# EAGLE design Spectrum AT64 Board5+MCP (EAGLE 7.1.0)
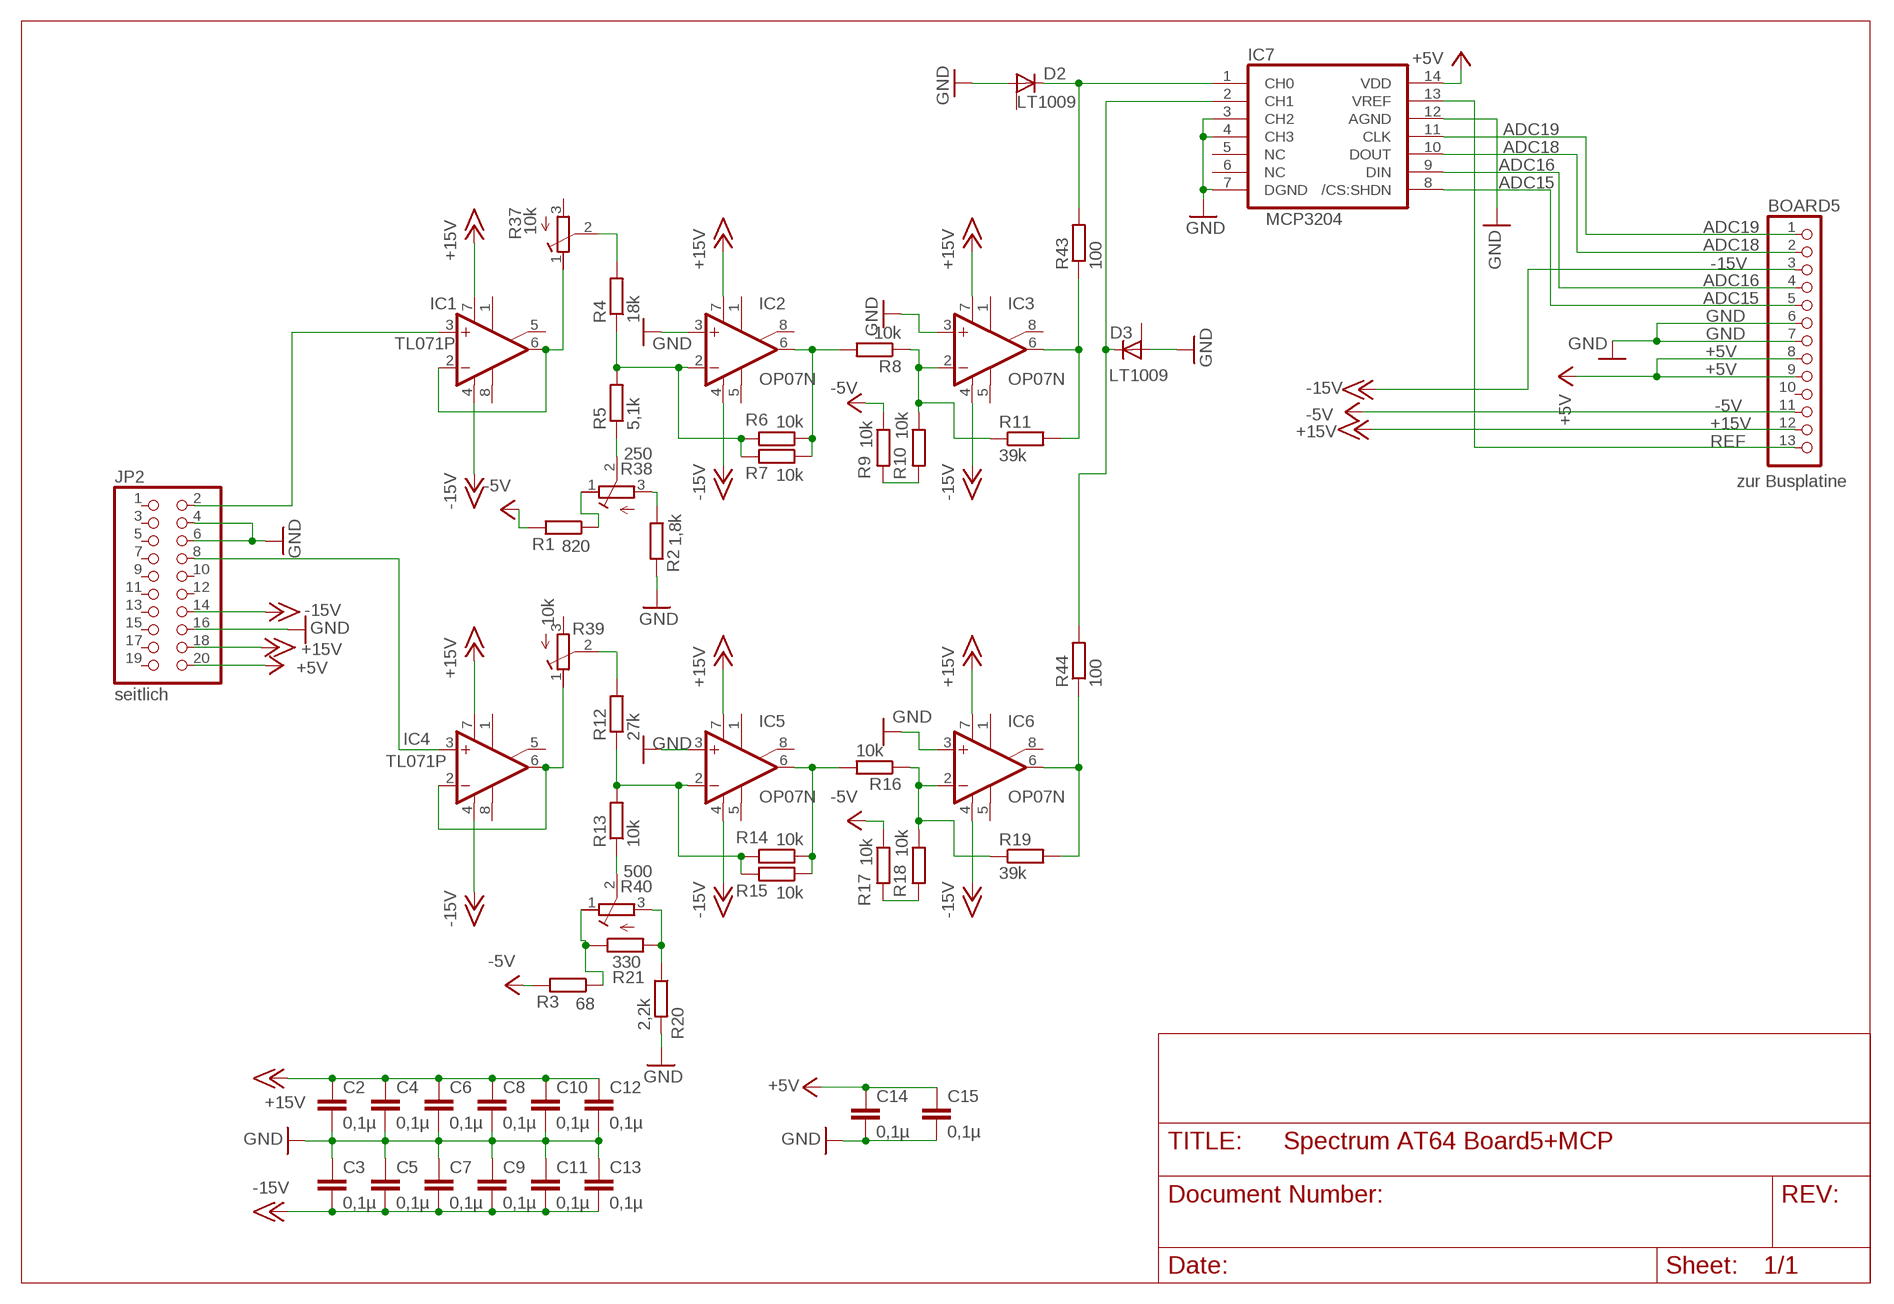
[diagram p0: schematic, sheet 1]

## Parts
BOARD5  zur Busplatine  PINHD-1X13_2.54-90°  [1X13/90]
C2  0,1µ  C-EU050-025X075  [C050-025X075]
C3  0,1µ  C-EUC0805  [C0805]
C4  0,1µ  C-EU050-025X075  [C050-025X075]
C5  0,1µ  C-EUC0805  [C0805]
C6  0,1µ  C-EU050-025X075  [C050-025X075]
C7  0,1µ  C-EU050-025X075  [C050-025X075]
C8  0,1µ  C-EU050-025X075  [C050-025X075]
C9  0,1µ  C-EU050-025X075  [C050-025X075]
C10  0,1µ  C-EU050-025X075  [C050-025X075]
C11  0,1µ  C-EU050-025X075  [C050-025X075]
C12  0,1µ  C-EU050-025X075  [C050-025X075]
C13  0,1µ  C-EU050-025X075  [C050-025X075]
C14  0,1µ  C-EU050-025X075  [C050-025X075]
C15  0,1µ  C-EU050-025X075  [C050-025X075]
D2  LT1009  [LT1009]
D3  LT1009  [LT1009]
IC1  TL071P  [DIL08]
IC2  OP07N  [DIL08]
IC3  OP07N  [DIL08]
IC4  TL071P  [DIL08]
IC5  OP07N  [DIL08]
IC6  OP07N  [DIL08]
IC7  MCP3204  [DIL14]
JP2  seitlich  PINHD-2X10_2.54-90°  [2X10/90]
R1  820  WIDERSTAND_10  [207.10]
R2  1,8k  WIDERSTAND_10  [207.10]
R3  68  WIDERSTAND_10  [207.10]
R4  18k  WIDERSTAND_10  [207.10]
R5  5,1k  WIDERSTAND_10  [207.10]
R6  10k  WIDERSTAND_10  [207.10]
R7  10k  WIDERSTAND_10  [207.10]
R8  10k  WIDERSTAND_10  [207.10]
R9  10k  WIDERSTAND_10  [207.10]
R10  10k  WIDERSTAND_10  [207.10]
R11  39k  WIDERSTAND_10  [207.10]
R12  27k  WIDERSTAND_10  [207.10]
R13  10k  WIDERSTAND_10  [207.10]
R14  10k  WIDERSTAND_10  [207.10]
R15  10k  WIDERSTAND_10  [207.10]
R16  10k  WIDERSTAND_10  [207.10]
R17  10k  WIDERSTAND_10  [207.10]
R18  10k  WIDERSTAND_10  [207.10]
R19  39k  WIDERSTAND_10  [207.10]
R20  2,2k  WIDERSTAND_10  [207.10]
R21  330  WIDERSTAND_10  [207.10]
R37  10k  R-TRIMM43P  [RTRIM43P]
R38  250  R-TRIMM43P  [RTRIM43P]
R39  10k  R-TRIMM43P  [RTRIM43P]
R40  500  R-TRIMM43P  [RTRIM43P]
R43  100  WIDERSTAND_10  [207.10]
R44  100  WIDERSTAND_10  [207.10]

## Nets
+5V: BOARD5.8 BOARD5.9 C14.1 C15.1 IC7.14(VDD) JP2.20
+15V: BOARD5.12 C2.1 C4.1 C6.1 C8.1 C10.1 C12.1 IC1.7(V+) IC2.7(V+) IC3.7(V+) IC4.7(V+) IC5.7(V+) IC6.7(V+) JP2.18
-5V: BOARD5.11 R1.2 R3.2 R9.1 R17.1
-15V: BOARD5.3 C3.2 C5.2 C7.2 C9.2 C11.2 C13.2 IC1.4(V-) IC2.4(V-) IC3.4(V-) IC4.4(V-) IC5.4(V-) IC6.4(V-) JP2.14
ADC15: BOARD5.5 IC7.8(/CS:SHDN)
ADC16: BOARD5.4 IC7.9(DIN)
ADC18: BOARD5.2 IC7.10(DOUT)
ADC19: BOARD5.1 IC7.11(CLK)
GND: BOARD5.6 BOARD5.7 C2.2 C3.1 C4.2 C5.1 C6.2 C7.1 C8.2 C9.1 C10.2 C11.1 C12.2 C13.1 C14.2 C15.2 D2.-(A) D3.-(A) IC2.3(+IN) IC3.3(+IN) IC5.3(+IN) IC6.3(+IN) IC7.3(CH2) IC7.4(CH3) IC7.7(DGND) IC7.12(AGND) JP2.4 JP2.6 JP2.16 R2.2 R20.2
N$1: R1.1 R38.1(A)
N$2: R2.1 R38.3(E)
N$3: R3.1 R21.1 R40.1(A)
N$4: R20.1 R21.2 R40.3(E)
N$6: IC1.3(+IN) JP2.2
N$7: IC1.2(-IN) IC1.6(OUT) R37.1(A)
N$8: R5.1 R38.2(S)
N$9: D3.+(C) IC7.2(CH1) R44.2
N$10: R4.2 R37.2(S)
N$11: IC2.6(OUT) R6.1 R7.1 R8.2
N$12: IC2.2(-IN) R4.1 R5.2 R6.2 R7.2
N$13: IC3.2(-IN) R8.1 R10.1 R11.1
N$14: R9.2 R10.2
N$15: IC3.6(OUT) R11.2 R43.1
N$16: IC4.3(+IN) JP2.8
N$17: D2.+(C) IC7.1(CH0) R43.2
N$18: IC4.2(-IN) IC4.6(OUT) R39.1(A)
N$19: R13.1 R40.2(S)
N$20: R12.2 R39.2(S)
N$21: IC5.6(OUT) R14.1 R15.1 R16.2
N$22: IC5.2(-IN) R12.1 R13.2 R14.2 R15.2
N$23: IC6.2(-IN) R16.1 R18.1 R19.1
N$24: R17.2 R18.2
N$25: IC6.6(OUT) R19.2 R44.1
REF: BOARD5.13 IC7.13(VREF)
Unconnected: BOARD5.10 D2.ADJ D3.ADJ IC1.1(ON1) IC1.5(ON2) IC1.8(OPT) IC2.1(ON1) IC2.5(OPT) IC2.8(ON2) IC3.1(ON1) IC3.5(OPT) IC3.8(ON2) IC4.1(ON1) IC4.5(ON2) IC4.8(OPT) IC5.1(ON1) IC5.5(OPT) IC5.8(ON2) IC6.1(ON1) IC6.5(OPT) IC6.8(ON2) IC7.5(NC) IC7.6(NC) JP2.1 JP2.3 JP2.5 JP2.7 JP2.9 JP2.10 JP2.11 JP2.12 JP2.13 JP2.15 JP2.17 JP2.19 R37.3(E) R39.3(E)

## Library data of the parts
BOARD5 = pinhead-2:PINHD-1X13: PIN HEADER
C2-C15 = rcl:C-EU: CAPACITOR, European symbol
D2 D3 = 1Eigene:LT1009
IC1 IC4 = linear:TL071: OP AMP
IC2 IC3 IC5 IC6 = linear:OP07*: OP AMP
IC7 = 1Eigene:MCP3204
JP2 = pinhead-2:PINHD-2X10: PIN HEADER
R1-R21 R43 R44 = 1Eigene:WIDERSTAND_10
R37-R40 = rcl:R-TRIMM: Trimm resistor

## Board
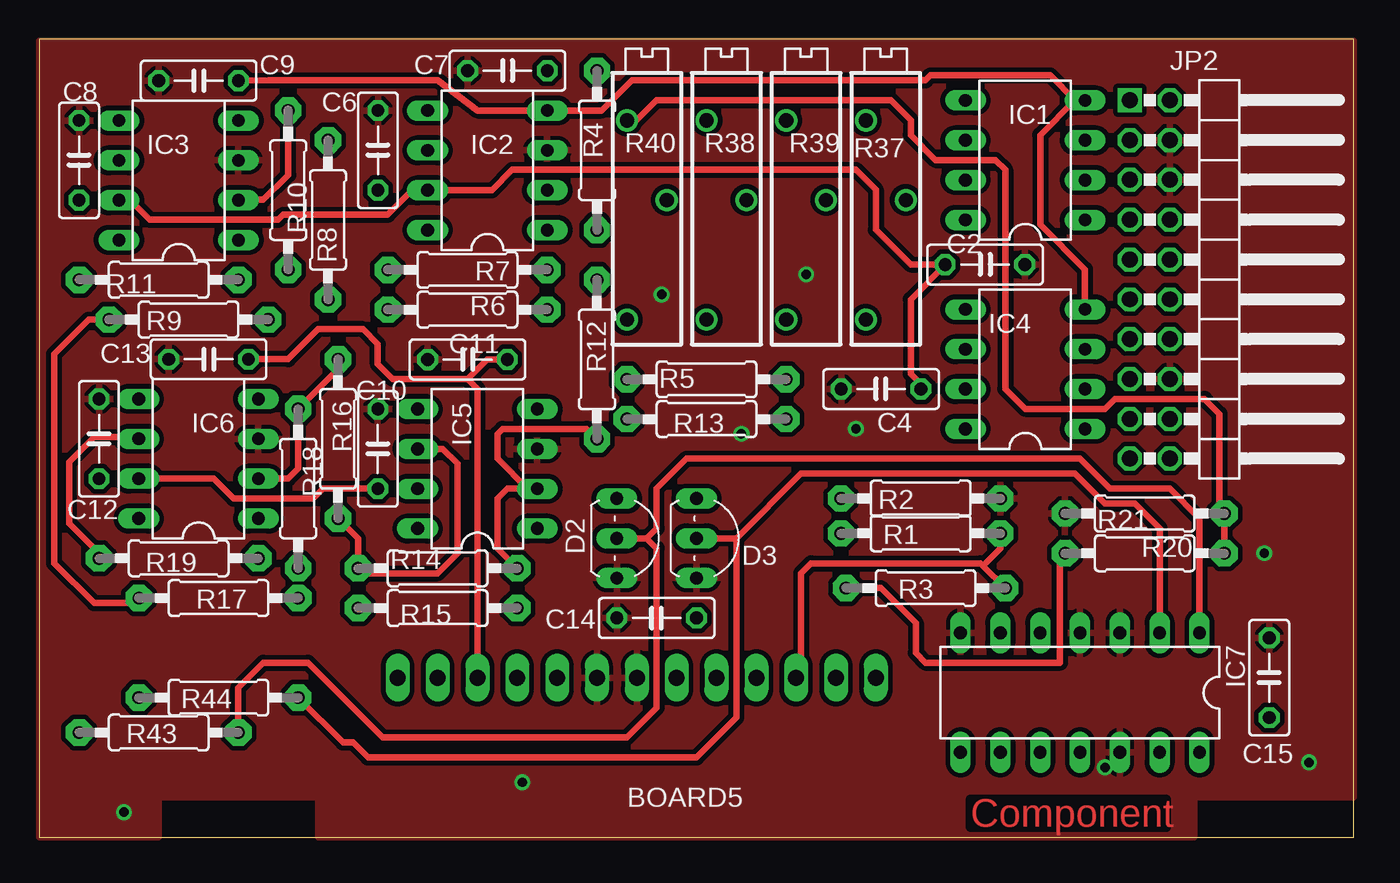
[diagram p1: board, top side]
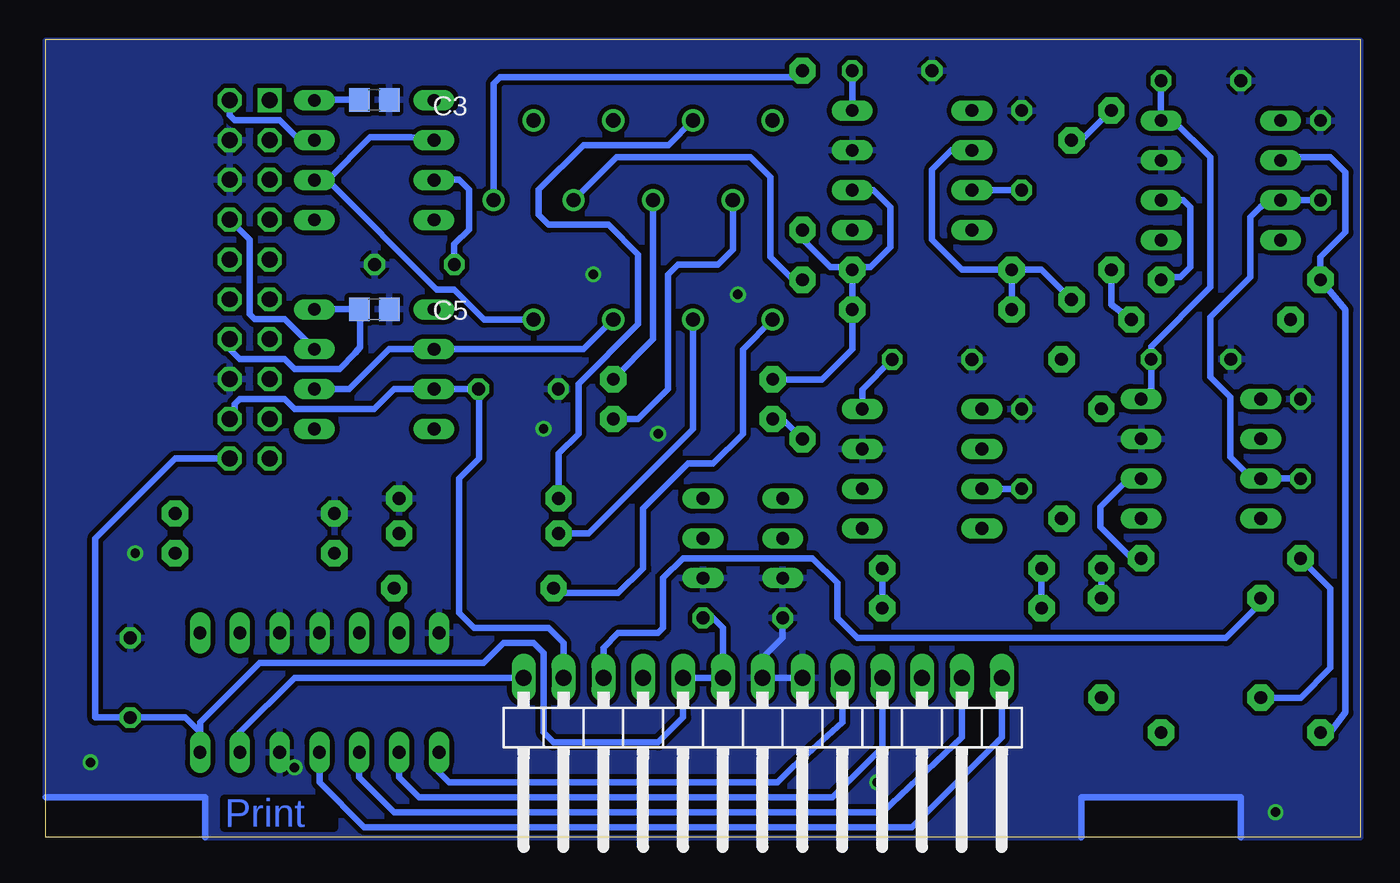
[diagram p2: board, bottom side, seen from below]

Size 83.8 x 50.88 mm. Coordinates in mm from the lower left corner, seen from the top.
Outline: 0,0 83.8,0 83.8,50.88 0,50.88 0,0
Copper layers (1*16): Top 0.035mm / dielectric 1.5mm / Bottom 0.035mm
Design rules "default *": minimum track width 0.4mm, minimum drill 0.6mm, track to track 0.3mm, track to pad 0.3mm, pad to pad 0.3mm, via to via 0.3mm, smd to smd 0.3mm, copper to edge 0mil, drill to drill 8mil, minimum pad ring 10mil, minimum via ring 8mil, stop-mask expansion 4mil, vias tented up to drill 0mil, thermal gap 10mil

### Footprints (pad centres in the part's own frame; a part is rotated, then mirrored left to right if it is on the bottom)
1X13/90 = drill 1.016 long: 1 -15.24,-3.81; 2 -12.7,-3.81; 3 -10.16,-3.81; 4 -7.62,-3.81; 5 -5.08,-3.81; 6 -2.54,-3.81; 7 0,-3.81; 8 2.54,-3.81; 9 5.08,-3.81; 10 7.62,-3.81; 11 10.16,-3.81; 12 12.7,-3.81; 13 15.24,-3.81
C050-025X075 = drill 0.813 octagon: 1 -2.54,0; 2 2.54,0
C0805 = smd 1.3 x 1.5: 1 -0.95,0; 2 0.95,0
LT1009 = drill 0.813 long: + 0,0; - 2.54,0; ADJ -2.54,0
DIL08 = drill 0.813 long: 1 -3.81,-3.81; 2 -1.27,-3.81; 3 1.27,-3.81; 4 3.81,-3.81; 5 3.81,3.81; 6 1.27,3.81; 7 -1.27,3.81; 8 -3.81,3.81
DIL14 = drill 0.813 long: 1 -6.35,-3.81; 2 -3.81,-3.81; 3 -1.27,-3.81; 4 1.27,-3.81; 5 3.81,-3.81; 6 6.35,-3.81; 7 8.89,-3.81; 8 8.89,3.81; 9 6.35,3.81; 10 3.81,3.81; 11 1.27,3.81; 12 -1.27,3.81; 13 -3.81,3.81; 14 -6.35,3.81
2X10/90 = drill 1.016 square: 1 -11.43,-6.35 | drill 1.016 octagon: 2 -11.43,-3.81; 3 -8.89,-6.35; 4 -8.89,-3.81; 5 -6.35,-6.35; 6 -6.35,-3.81; 7 -3.81,-6.35; 8 -3.81,-3.81; 9 -1.27,-6.35; 10 -1.27,-3.81; 11 1.27,-6.35; 12 1.27,-3.81; 13 3.81,-6.35; 14 3.81,-3.81; 15 6.35,-6.35; 16 6.35,-3.81; 17 8.89,-6.35; 18 8.89,-3.81; 19 11.43,-6.35; 20 11.43,-3.81
207.10 = drill 0.813 pad 1.676 octagon: 1 -5.08,0; 2 5.08,0
RTRIM43P = drill 0.9: 1 -7.62,1.27; 2 0,-1.27; 3 5.08,1.27

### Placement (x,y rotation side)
BOARD5  38.1,6.35 180 bottom
C2  60.31,36.51 0 top
C3  62.86,47.01 180 bottom
C4  53.68,28.57 180 top
C5  62.86,33.66 180 bottom
C6  21.59,43.79 90 top
C7  29.85,48.87 0 top
C8  2.54,43.15 90 top
C9  10.16,48.23 0 top
C10  21.59,24.75 90 top
C11  27.31,30.46 0 top
C12  3.81,25.39 90 top
C13  10.79,30.47 0 top
C14  39.37,13.97 180 top
C15  78.42,10.16 90 top
D2  36.83,19.05 270 top
D3  41.91,19.05 270 top
IC1  62.87,43.16 90 top
IC2  28.58,42.52 90 top
IC3  8.89,41.88 90 top
IC4  62.87,29.84 90 top
IC5  27.94,23.48 90 top
IC6  10.16,24.12 90 top
IC7  67.63,9.21 180 top
JP2  75.88,35.56 270 top
R1  56.2,19.37 0 top
R2  56.2,21.59 0 top
R3  56.52,15.88 0 top
R4  35.56,43.79 90 top
R5  42.55,29.19 180 top
R6  27.31,33.63 0 top
R7  27.31,36.17 0 top
R8  18.41,39.35 270 top
R9  9.52,33 0 top
R10  15.87,41.26 270 top
R11  7.62,35.54 180 top
R12  35.56,30.46 90 top
R13  42.55,26.65 180 top
R14  25.4,17.14 0 top
R15  25.4,14.6 0 top
R16  19.05,25.39 270 top
R17  11.44,15.24 0 top
R18  16.51,22.23 270 top
R19  8.89,17.77 180 top
R20  70.48,20.64 180 top
R21  70.48,18.1 0 top
R37  53.98,40.62 90 top
R38  43.82,40.62 90 top
R39  48.9,40.62 90 top
R40  38.74,40.62 90 top
R43  7.62,6.67 0 top
R44  11.43,8.89 0 top

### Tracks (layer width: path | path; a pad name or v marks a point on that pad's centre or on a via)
+5V
  Bottom 0.406: C14.1 41.27,13.97 40.64,13.34 BOARD5.8 BOARD5.9 43.18,7.62 44.77,6.03 51.44,6.03 52.07,6.67 52.07,11.75 52.7,12.38 54.61,12.38 55.88,11.11 70.17,11.11 73.98,7.3 73.98,6.67 | IC7.14 73.98,6.67 | JP2.20 75.56,24.13 80.64,19.05 80.64,7.62 C15.1 74.93,7.62 73.98,6.67
+15V
  Top 0.406: IC3.7 5.16,40.54 5.88,40.54 7.05,39.37 15.24,39.37 15.56,39.69 22.23,39.69 23.79,41.25 IC2.7 28.87,41.25 30.16,42.55 52.07,42.55 53.34,41.27 53.34,38.73 55.56,36.51 C2.1 57.79,36.52 55.56,34.29 55.56,29.53 56.52,28.57 C4.1 | IC6.7 11.12,22.86 12.38,21.59 17.46,21.59 18.1,22.23 21.57,22.23 C10.1
  Bottom 0.406: C10.1 23.49,22.21 IC5.7 | C12.1 IC6.7 6.92,22.86 8.29,24.23 8.29,28.05 9.56,29.33 9.56,33.15 7.01,35.7 7.01,39.53 6.38,40.16 5.53,40.8 IC3.7 3.81,40.62 C8.1 | IC2.7 C6.1 | 60.34,28.57 61.59,28.57 62.87,27.3 67.94,27.3 68.58,27.94 71.44,27.94 71.75,27.62 71.75,26.99 JP2.18 | 60.34,28.57 IC4.7 | 60.34,28.57 C4.1 56.2,28.55 56.2,24.13 57.47,22.86 57.47,14.29 56.52,13.34 51.75,13.34 50.8,12.38 BOARD5.12 | C2.1 57.77,37.8 56.83,38.73 56.83,41.27 57.47,41.91 59.04,41.91 IC1.7
-5V
  Top 0.406: R9.1 3.15,33 0.95,30.8 0.95,17.46 3.49,14.92 6.04,14.92 R17.1 | BOARD5.11 48.58,10.48 48.58,16.83 49.21,17.46 60.01,17.46 60.17,17.3 | 60.17,17.3 R3.2 | R1.2 61.28,18.41 60.17,17.3
  Bottom 0.406: R17.1 6.36,14.92 8.57,12.7 32.07,12.7 33.34,13.97 33.34,16.19 34.92,17.78 43.18,17.78 44.45,16.51 44.45,13.34 44.77,13.02 47.31,13.02 48.26,12.06 BOARD5.11
-15V
  Top 0.406: C9.2 14.63,48.26 25.4,48.26 27.96,46.33 IC2.4 35.85,46.33 37.78,48.26 56.52,48.26 56.83,48.58 64.45,48.58 66.04,46.99 | C11.2 28.55,30.46 27.3,29.21 | 27.3,29.21 22.54,29.21 21.59,30.16 21.59,31.43 20.64,32.38 17.78,32.38 15.88,30.48 C13.2 | IC4.4 66.68,36.19 63.82,39.05 63.82,44.77 66.04,46.99 | 66.04,46.99 66.66,46.99 IC1.4 | BOARD5.3 27.94,28.57 27.3,29.21
  Bottom 0.406: 13.85,28.05 IC6.4 13.34,28.57 C13.2 13.34,31.29 9.56,35.06 9.56,43.35 11.9,45.7 IC3.4 C9.2 | IC2.4 C7.2 | 66.8,33.65 IC4.4 66.66,33.66 C5.2 63.76,33.61 63.76,31.24 64.08,30.86 65.09,29.84 67.94,29.84 68.58,30.48 71.44,30.48 72.07,31.11 JP2.14 | IC5.4 31.75,28.55 C11.2 | C3.2 66.64,47.01 IC1.4
ADC15
  Bottom 0.406: BOARD5.5 33.02,7.3 36.2,4.45 37.15,3.49 58.1,3.49 58.74,4.13 IC7.8
ADC16
  Bottom 0.406: BOARD5.4 30.48,5.71 33.66,2.54 60.01,2.54 61.28,3.81 IC7.9
ADC18
  Bottom 0.406: BOARD5.2 25.4,6.35 30.48,1.59 61.59,1.59 63.82,3.81 IC7.10
ADC19
  Bottom 0.406: BOARD5.1 22.86,6.35 28.57,0.64 63.5,0.64 66.36,3.49 IC7.11
GND  (via drill 0.6, 0.6 pad 1.02)
  Bottom 0.406: BOARD5.6 BOARD5.7 38.1,11.43 36.83,12.7 C14.2 | 7.62,0 7.62,2.54 17.78,2.54 17.78,0 | 83.82,2.54 73.66,2.54 73.66,0
  other vias: 48.9,35.88 52.07,26.04 80.96,4.76 78.11,18.1 67.94,4.45 5.4,1.59 39.69,34.61 30.8,3.49 44.77,25.72
  pour Top: 0,50.78 83.82,50.78 83.82,2.54 73.66,2.54 73.66,0 17.78,0 17.78,2.54 7.62,2.54 7.62,0 0,0
  pour Bottom: 0,0 0,50.78 83.82,50.78 83.82,2.54 73.66,2.54 73.66,0 17.78,0 17.78,2.54 7.62,2.54 7.62,0
N$1
  Bottom 0.406: R38.1 42.55,26.04 49.21,19.37 R1.1
N$2
  Bottom 0.406: R38.3 44.12,44.13 49.53,44.13 52.39,41.27 52.39,39.69 51.75,39.05 47.94,39.05 46.04,37.15 46.04,32.7 49.85,28.89 49.85,25.72 51.12,24.45 R2.1
N$3
  Top 0.406: R3.1 53.66,15.88 55.88,13.65 55.88,11.75 56.52,11.11 65.09,11.11 65.09,17.78 R21.1
  Bottom 0.406: R40.1 39.37,31.1 39.37,25.72 41.27,23.81 42.86,23.81 45.72,20.95 45.72,17.14 47.31,15.56 51.12,15.56 R3.1
N$4
  Top 0.406: R40.3 38.08,45.7 39.37,46.99 54.29,46.99 55.56,45.72 55.56,44.77 57.15,43.18 60.96,43.18 61.59,42.55 61.59,28.57 62.87,27.3 67.94,27.3 68.58,27.94 74.3,27.94 75.25,26.99 75.25,20.95 R20.1 R21.2
N$6
  Bottom 0.406: IC1.3 67.61,44.44 68.9,45.72 71.75,45.72 72.07,46.04 JP2.2
N$7
  Bottom 0.406: 65.85,41.9 IC1.2 | 65.85,41.9 63.12,44.63 60.52,44.63 IC1.6 | R37.1 55.86,33 57.78,34.92 58.88,34.92 65.85,41.9
N$8
  Bottom 0.406: R5.1 47.62,29.21 45.09,31.75 R38.2
N$9
  Top 0.406: 44.45,19.05 44.45,7.62 41.91,5.08 20.95,5.08 20,6.03 19.37,6.03 R44.2 | 44.45,19.05 D3.+ | IC7.2 71.44,19.68 69.85,21.27 67.94,21.27 66.04,23.18 48.58,23.18 44.45,19.05
N$10
  Bottom 0.406: R37.2 55.25,48.03 54.83,48.45 35.98,48.45 R4.2
N$11
  Bottom 0.406: R8.2 20.32,36.18 R7.1 | R7.1 R6.1 | IC2.6 26.06,43.79 27.3,42.55 27.3,38.1 25.4,36.2 22.25,36.2 R7.1
N$12
  Bottom 0.406: IC2.2 31.05,41.25 29.96,40.16 29.96,37.62 31.24,36.34 32.22,36.34 R7.2 | R7.2 R6.2 32.38,31.11 34.31,29.19 R5.2 | R4.1 35.56,38.12 33.79,36.34 32.55,36.34 R7.2
N$13
  Top 0.406: R10.1 15.87,42.23 14.29,40.64 12.72,40.64 IC3.2
  Bottom 0.406: R8.1 17.78,44.43 R10.1 | IC3.2 11.29,40.62 10.84,40.16 10.84,36.34 11.48,35.7 12.54,35.7 R11.1
N$14
  Bottom 0.406: R10.2 15.87,33.95 R9.2
N$15
  Bottom 0.406: R43.1 1.91,6.67 0.95,7.94 0.95,33.63 R11.2 2.54,36.99 0.95,38.57 0.95,42.4 1.91,43.35 3.19,43.35 4.88,43.35 IC3.6
N$16
  Bottom 0.406: IC4.3 68.58,33.02 70.48,33.02 70.8,33.34 70.8,38.1 JP2.8
N$17
  Top 0.406: 38.73,19.05 39.37,18.41 39.37,8.26 37.47,6.35 21.91,6.35 17.14,11.11 14.29,11.11 12.7,9.53 R43.2 | 38.73,19.05 D2.+ | 38.73,19.05 39.37,19.68 39.37,22.23 41.27,24.13 66.36,24.13 68.26,22.23 72.07,22.23 73.98,20.32 IC7.1
N$18
  Bottom 0.406: IC4.2 64.46,28.57 61.91,31.11 60.34,31.11 IC4.6 49.52,31.11 R39.1
N$19
  Bottom 0.406: R13.1 46.05,26.66 44.13,28.57 44.13,35.88 43.5,36.51 40.96,36.51 40.01,37.47 R40.2
N$20
  Bottom 0.406: R12.2 36.17,35.54 37.62,36.98 37.62,42.08 38.89,43.35 47.43,43.35 R39.2
N$21
  Top 0.406: IC5.6 25.73,24.75 26.67,23.81 26.67,18.1 25.4,16.83 20.63,16.83 R14.1 20.32,19.04 R16.2
  Bottom 0.406: R15.1 R14.1
N$22
  Top 0.406: R14.2 29.21,18.41 29.21,21.59 29.84,22.23 31.74,22.23 IC5.2 31.13,22.21 29.21,24.13 29.21,25.72 29.53,26.04 34.91,26.04 R12.1
  Bottom 0.406: R15.2 R14.2 | R13.2 36.84,26.66 R12.1
N$23
  Top 0.406: R16.1 19.05,29.84 R18.1 16.51,23.5 15.88,22.86 IC6.2
  Bottom 0.406: IC6.2 14.76,22.86 16.58,21.04 16.58,19.76 14.66,17.85 14.05,17.85 R19.1
N$24
  Bottom 0.406: R17.2 R18.2
N$25
  Top 0.406: R19.2 3.81,18.1 1.91,20 1.91,23.91 3.49,25.5 6.24,25.5 IC6.6
  Bottom 0.406: R44.1 3.81,8.89 1.91,10.79 1.91,15.87 R19.2 | IC6.6 6.24,25.5
REF
  Bottom 0.406: BOARD5.13 67.94,10.16 71.44,6.67 IC7.13

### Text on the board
Top: Component
Bottom: Print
